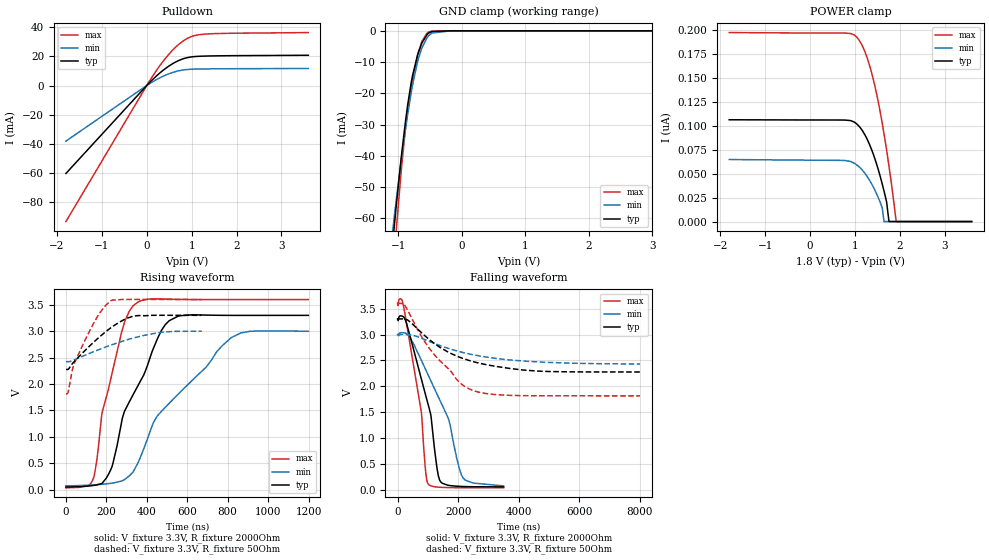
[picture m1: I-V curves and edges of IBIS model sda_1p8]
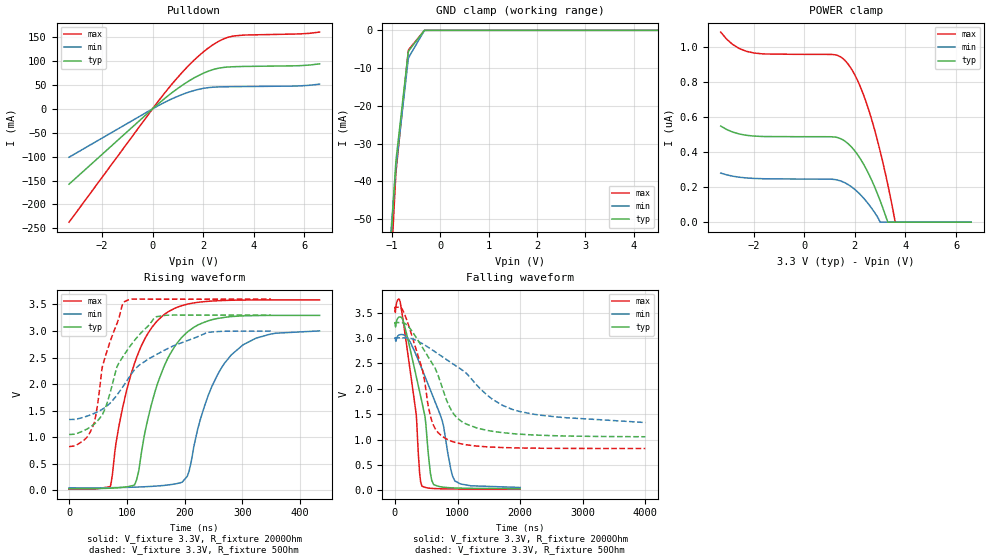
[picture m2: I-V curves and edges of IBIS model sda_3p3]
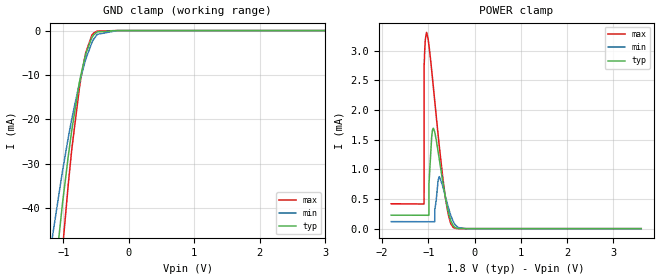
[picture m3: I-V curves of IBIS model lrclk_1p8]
|Texas Instruments Incorporated
| 2X50W/4Ohm PurePathTH Smart Amp
| Marketing part#   Voltage Range(Digital)   Package-type   #pins
| TAS5766MDCA   1.62V-3.6V   TSSOP   48
[IBIS Ver]   4.1
[File name]   tas5766m.ibs
[File Rev]   1.1
[Date]   01/23/2014
[Source]
| Texas Instruments Incorporated.
| Analog-eLab Design Center, HPA
| 12500 TI Blvd
| Dallas, TX -75243
[Notes]   Revision History:
| Rev 1.1: 01/23/2014
| - Updated ADR1 and ADR2 models
| Rev 1.0: 10/03/2013
| - Initial version of the model
| - Model generated from simulations in TISPICE
| - Model matched to SPICE simulation
| - Model names with a sda_1p8,lrclk_1p8,adr*_1p8 contain the models
|   for 1.8V (1.62V and 1.98V) operation.All other Model names with a trailing
|   _1p8 contains the model for 1.8V (1.65V and 1.95V) operation.
|   Model names with trailing _3p3contains the model for
|   3.3V (3.0V and 3.6V) operation.
| - Combined Pulldown/up non-monotonicity warnings for GPIO6_xxxx,
|   GPIO_xxxx. LRCK_xxxx reflect simulation results and can
|   safely ignored.
| - C_comp although listed in numerical order of value are
|   obtained from varying PVT conditions. For PVT conditions for
|   each specific value refer the buffer description under
|   respective [Model]. IBIS model user is responsible for using
|   appropriate C_comp to simulate for Signal Integrity.
|*EXCEPTION:   *
|* - For SDA and ADR2 models,There will be small leakage currents in   *
|* - POWER clamp IV-table because of the resistor (RES3T_NWELL) connected   *
|* - to the pad.   *
[Disclaimer]
| This model is designed as an aid for customers of Texas Instruments.
| TI and its licensors and suppliers make no warranties, either expressed
| or implied, with respect to this  model, including the warranties of
| merchantability or fitness for a particular purpose. The model is
| provided solely on an "as is" basis. The entire risk as to its quality
| and performance is with the customer.
[Copyright]
(C) Copyright 2014 Texas Instruments Incorporated.All rights reserved.
|   TAS5766MDCA
[Component]   TAS5766MDCA
[Manufacturer]   TI
[Package]   |48 TSSOP  -   package
|   typ   min   max
R_pkg   0.1   0.08   0.12
L_pkg   1.5nH   1.35nH   1.65nH
C_pkg   0.5pF   0.4pF   0.6pF
[Pin]  signal_name   model_name   R_pin   L_pin   C_pin
1   BSNR   NC   NA   NA   NA
2   OUTNR   NC   NA   NA   NA
3   GND   GND   NA   NA   NA
4   OUTPR   NC   NA   NA   NA
5   BSPR   NC   NA   NA   NA
6   PVCC   POWER   NA   NA   NA
7   PVCC   POWER   NA   NA   NA
8   GVDD   NC   NA   NA   NA
9   GAIN/FSW   NC   NA   NA   NA
10   GND   GND   NA   NA   NA
11   INNR   NC   NA   NA   NA
12   INPR   NC   NA   NA   NA
13   DACR   NC   NA   NA   NA
14   AVDD   POWER   NA   NA   NA
15   GND   GND   NA   NA   NA
16   SDA   SDA   NA   NA   NA
17   SCL   MC   NA   NA   NA
18   GPIO1   GPIO   NA   NA   NA
19   GPIO2   GPIO   NA   NA   NA
20   ADR2   ADR2   NA   NA   NA
21   GPIO3   GPIO6   NA   NA   NA
22   SCLK   SCK_IN   NA   NA   NA
23   BCLK   BCK_IN   NA   NA   NA
24   DIN   SCK_IN   NA   NA   NA
25   LRCLK   LRCLK   NA   NA   NA
26   ADR1   ADR1   NA   NA   NA
27   XSMT/UVP   DEMP_IN   NA   NA   NA
28   LDOO   NC   NA   NA   NA
29   GND   GND   NA   NA   NA
30   DVDD   POWER   NA   NA   NA
31   CPVDD   POWER   NA   NA   NA
32   CAPP   NC   NA   NA   NA
33   GND   GND   NA   NA   NA
34   CAPM   NC   NA   NA   NA
35   VNEG   NC   NA   NA   NA
36   DACL   NC   NA   NA   NA
37   INPL   NC   NA   NA   NA
38   INNL   NC   NA   NA   NA
39   GND   GND   NA   NA   NA
40   /FAULTZ   NC   NA   NA   NA
41   AVCC   POWER   NA   NA   NA
42   PVCC   POWER   NA   NA   NA
43   PVCC   POWER   NA   NA   NA
44   BSPL   NC   NA   NA   NA
45   OUTPL   NC   NA   NA   NA
46   GND   GND   NA   NA   NA
47   OUTNL   NC   NA   NA   NA
48   BSNL   NC   NA   NA   NA
|   Model Selectors
[Model Selector] SDA
sda_3p3   3.3V digital I/O_open_drain
sda_1p8   1.8V digital I/O_open_drain
[Model Selector] LRCLK
lrclk_3p3   3.3V digital input
lrclk_1p8   1.8V digital input
[Model Selector] ADR1
adr1_3p3   3.3V digital input
adr1_1p8   1.8V digital input
[Model Selector] ADR2
adr2_3p3   3.3V digital input
adr2_1p8   1.8V digital input
[Model Selector] MC
mc_3p3   3.3V digital input
mc_1p8   1.8V digital input
[Model Selector] GPIO
gpio_3p3   3.3V digital I/O
gpio_1p8   1.8V digital I/O
[Model Selector] GPIO6
gpio6_3p3   3.3V digital I/O
gpio6_1p8   1.8V digital I/O
[Model Selector] BCK_IN
bck_in_3p3   3.3V digital input
bck_in_1p8   1.8V digital input
[Model Selector] DEMP_IN
demp_in_3p3   3.3V digital input
demp_in_1p8   1.8V digital input
[Model Selector] FLT_IN
flt_in_3p3   3.3V digital input
flt_in_1p8   1.8V digital input
[Model Selector] SCK_IN
sck_in_3p3   3.3V digital input
sck_in_1p8   1.8V digital input
| Models and submodels in the file (22): sda_1p8 (I/O_open_drain), sda_3p3 (I/O_open_drain), lrclk_1p8 (Input), lrclk_3p3 (Input), adr1_1p8 (Input), adr1_3p3 (Input), adr2_1p8 (Input), adr2_3p3 (Input), mc_1p8 (Input), mc_3p3 (Input), gpio_1p8 (I/O), gpio_3p3 (I/O), gpio6_1p8 (I/O), gpio6_3p3 (I/O), bck_in_1p8 (Input), bck_in_3p3 (Input), demp_in_1p8 (Input), demp_in_3p3 (Input), flt_in_1p8 (Input), flt_in_3p3 (Input), sck_in_1p8 (Input), sck_in_3p3 (Input)
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|   sda_1p8 Model
[Model]   sda_1p8
Model_type   I/O_open_drain
Polarity   Non-Inverting
Vinl = 0.54
Vinh = 1.26
Vmeas = 0.9
Vref = 1.8
Cref = 400pF
Rref = 2000
|   typ   min   max
|   (nom PVT)   (fast PVT)   (slow PVT)
C_comp   1.016e-11   1.003e-11   1.042e-11
[Model spec]
|subparameter
Vinl   0.54   0.486   0.594
Vinh   1.26   1.134   1.386
| Where nom  PVT is Nominal Process, 1.8V, 27C
|   Fast PVT is Strong Process,  1.98V, -40C
|   Slow PVT is Weak Process,   1.62V, 125C
[Voltage Range]   1.8   1.62   1.98
|Junction Temperature
[Temperature Range]   27   125   -40
[Pullup Reference]   1.8   1.62   1.98
[Pulldown Reference]   0   0   0
[Power Clamp Reference]   1.8   1.62   1.98
[GND Clamp Reference]   0   0   0
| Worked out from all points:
|   slope of the pulldown table from 0 to 0.27 V, typ, clamps not added: 33.8 ohm
|   GND clamp passes 1 mA (typ) near -0.54 V on its own axis
|   falling waveform, V_fixture 3.3V, R_fixture 2000Ohm: 20-80 % time 682ns typ, 1.08us min, 481ns max; typ from 3.3 V to 0.054 V
|   rising waveform, V_fixture 3.3V, R_fixture 2000Ohm: 20-80 % time 185ns typ, 339ns min, 111ns max; typ from 0.051 V to 3.3 V
|   falling waveform, V_fixture 3.3V, R_fixture 50Ohm: 20-80 % time 1.78us typ, 2.22us min, 1.37us max; typ from 3.3 V to 2.28 V
|   rising waveform, V_fixture 3.3V, R_fixture 50Ohm: 20-80 % time 179ns typ, 257ns min, 124ns max; typ from 2.27 V to 3.3 V
[Pulldown]
|   Voltage   I(typ)   I(min)   I(max)
-1.8V     -60.2mA    -38.06mA   -93.14mA
113.4mV   3.549mA    2.205mA    5.58mA
290.9mV   8.545mA    5.245mA    13.57mA
466.2mV   12.73mA    7.698mA    20.46mA
597.4mV   15.29mA    9.13mA     24.88mA
790.2mV   18.06mA    10.53mA    30.04mA
1.022V    19.67mA    11.17mA    33.79mA
1.328V    20.17mA    11.36mA    35.25mA
3.6V      20.7mA     11.65mA    36.23mA
[GND Clamp]
|   Voltage   I(typ)   I(min)   I(max)
-1.8V     -334.9mA   -249.2mA   -436.8mA
-1.252V   -106.9mA   -94.42mA   -128.4mA
-1.061V   -62.46mA   -59.36mA   -71.93mA
-1.028V   -55.6mA    -53.82mA   -63.33mA
-943.2mV  -39.01mA   -40.16mA   -42.95mA
-880.3mV  -28.25mA   -30.88mA   -30.48mA
-795.8mV  -16.72mA   -19.9mA    -18.15mA
-696mV    -7.878mA   -9.987mA   -8.008mA
-627.4mV  -3.937mA   -5.498mA   -3.416mA
-518.4mV  -696.6uA   -1.541mA   -348.2uA
-180mV    -66.44nA   -964.8nA   -76.84nA
3.6V      0A         0A         0A
[POWER Clamp]
|   Voltage   I(typ)   I(min)   I(max)
-1.8V     106.1nA    64.68nA    197nA
732.5mV   105.9nA    63.75nA    196.5nA
1.004V    103.1nA    60.33nA    193.9nA
1.222V    90.44nA    50.33nA    177.2nA
1.328V    80.07nA    42.88nA    162.4nA
1.449V    64.89nA    32.34nA    140.4nA
1.607V    39.39nA    14.45nA    102.8nA
1.649V    31.66nA    0A         91.34nA
1.706V    20.31nA    0A         74.4nA
1.758V    0A         0A         57.99nA
1.919V    0A         0A         0A
3.6V      0A         0A         0A
[Ramp]
R_load = 2000
|   typ   min   max
dV/dt_r   1.94882/1.84537e-07   1.7551/3.39722e-07   2.13774/1.10149e-07
dV/dt_f   1.94589/6.79836e-07   1.72347/1.07088e-06   2.13801/4.80512e-07
[Falling Waveform]
V_fixture = 3.3V
V_fixture_min = 3V
V_fixture_max = 3.6V
R_fixture = 2000Ohm
|   Time   V(typ)   V(min)   V(max)
0s        3.3V       3V         3.6V
147.6ns   3.357V     3.036V     3.663V
300ns     3.202V     3.017V     3.201V
788.1ns   2.131V     2.498V     1.48V
908.8ns   1.865V     2.344V     456.9mV
996.5ns   1.673V     2.233V     121.6mV
1.419us   152.5mV    1.701V     45.98mV
1.684us   83.95mV    1.36V      40.46mV
2.172us   61.38mV    218.6mV    37.06mV
3.5us     54.21mV    73.33mV    35.56mV
[Rising Waveform]
V_fixture = 3.3V
V_fixture_min = 3V
V_fixture_max = 3.6V
R_fixture = 2000Ohm
|   Time   V(typ)   V(min)   V(max)
0s        50.87mV    74.1mV     35.46mV
135.6ns   80.3mV     91.04mV    212.9mV
178.9ns   122.3mV    103mV      1.462V
227.5ns   432.9mV    124mV      2.196V
279.8ns   1.365V     171.3mV    3.04V
335.8ns   1.824V     360.7mV    3.492V
472.6ns   3.016V     1.484V     3.609V
552.3ns   3.279V     1.796V     3.6V
864.3ns   3.298V     2.965V     3.597V
1.199us   3.299V     2.999V     3.598V
[Falling Waveform]
V_fixture = 3.3V
V_fixture_min = 3V
V_fixture_max = 3.6V
R_fixture = 50Ohm
|   Time   V(typ)   V(min)   V(max)
0s        3.3V       3V         3.6V
239.2ns   3.299V     3.001V     3.564V
801ns     3.029V     2.925V     2.951V
1.231us   2.82V      2.824V     2.597V
1.755us   2.636V     2.717V     2.29V
2.045us   2.562V     2.669V     2.074V
2.464us   2.48V      2.612V     1.923V
3.198us   2.388V     2.542V     1.84V
4.609us   2.294V     2.471V     1.816V
8us       2.276V     2.428V     1.814V
[Rising Waveform]
V_fixture = 3.3V
V_fixture_min = 3V
V_fixture_max = 3.6V
R_fixture = 50Ohm
|   Time   V(typ)   V(min)   V(max)
0s        2.275V     2.423V     1.814V
10.75ns   2.277V     2.423V     1.848V
31.25ns   2.383V     2.44V      2.259V
40.5ns    2.422V     2.455V     2.387V
87.75ns   2.609V     2.534V     2.776V
155.8ns   2.856V     2.64V      3.275V
219.5ns   3.057V     2.732V     3.571V
346.3ns   3.291V     2.883V     3.6V
480.5ns   3.3V       2.981V     3.6V
671.3ns   3.3V       3V         3.6V
|   sda_3p3 Model
[Model]   sda_3p3
Model_type   I/O_open_drain
Polarity   Non-Inverting
Vinl = 0.8
Vinh = 2
Vmeas = 1.65
Vref = 3.3
Cref = 400pF
Rref = 2000
|   typ   min   max
|   (nom PVT)   (fast PVT)   (slow PVT)
C_comp   9.904e-12   9.904e-12   1.003e-11
| Where nom  PVT is Nominal Process, 3.3V, 27C
|   Fast PVT is Strong Process,  3.6V, -40C
|   Slow PVT is Weak Process,   3V, 125C
[Voltage Range]   3.3   3   3.6
|Junction Temperature
[Temperature Range]   27   125   -40
[Pullup Reference]   3.3   3   3.6
[Pulldown Reference]   0   0   0
[Power Clamp Reference]   3.3   3   3.6
[GND Clamp Reference]   0   0   0
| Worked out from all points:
|   slope of the pulldown table from 0 to 0.495 V, typ, clamps not added: 22.1 ohm
|   falling waveform, V_fixture 3.3V, R_fixture 2000Ohm: 20-80 % time 268ns typ, 434ns min, 189ns max; typ from 3.3 V to 0.036 V
|   rising waveform, V_fixture 3.3V, R_fixture 2000Ohm: 20-80 % time 54.2ns typ, 57.3ns min, 52.8ns max; typ from 0.035 V to 3.29 V
|   falling waveform, V_fixture 3.3V, R_fixture 50Ohm: 20-80 % time 518ns typ, 1.02us min, 316ns max; typ from 3.3 V to 1.06 V
|   rising waveform, V_fixture 3.3V, R_fixture 50Ohm: 20-80 % time 54.4ns typ, 96.8ns min, 33.8ns max; typ from 1.05 V to 3.3 V
[Pulldown]
|   Voltage   I(typ)   I(min)   I(max)
-3.3V     -157.6mA   -101.2mA   -237.1mA
459mV     20.85mA    13.12mA    31.8mA
897mV     38.95mA    24.09mA    59.96mA
1.434V    58.29mA    35.03mA    91.05mA
2.172V    78.17mA    44.18mA    126mA
2.442V    82.93mA    45.46mA    136mA
2.806V    86.68mA    46.14mA    146.3mA
3.231V    88.2mA     46.48mA    152.6mA
5.625V    90.03mA    47.68mA    156.5mA
6.6V      94.16mA    51.61mA    160.6mA
[GND Clamp]
|   Voltage   I(typ)   I(min)   I(max)
-3.3V     -1.594A    -1.313A    -1.903A
-1.104V   -71.9mA    -66.9mA    -83.83mA
-927mV    -36.1mA    -37.7mA    -39.48mA
-916.8mV  -34.31mA   -36.17mA   -37.38mA
-666.6mV  -6.007mA   -7.839mA   -5.788mA
-657.6mV  -5.489mA   -7.251mA   -5.183mA
-330mV    -4.474uA   -40.92uA   -707.9nA
6.6V      0A         0A         0A
[POWER Clamp]
|   Voltage   I(typ)   I(min)   I(max)
-3.3V     548.4nA    280.3nA    1.085uA
-2.828V   514.4nA    262.6nA    1.014uA
-1.986V   491.3nA    249.7nA    965.5nA
1.096V    487.3nA    245.1nA    957nA
1.53V     469.6nA    230.1nA    933.6nA
2.046V    397.8nA    181.1nA    827.2nA
2.303V    341.4nA    144.3nA    741.6nA
2.571V    268.7nA    97.75nA    630.3nA
3.003V    121.8nA    0A         404.4nA
3.303V    0A         0A         214.2nA
3.598V    0A         0A         0A
6.6V      0A         0A         0A
[Ramp]
R_load = 2000
|   typ   min   max
dV/dt_r   1.95666/5.39715e-08   1.76885/5.68771e-08   2.14112/5.31045e-08
dV/dt_f   1.9577/2.68023e-07   1.7646/4.3247e-07   2.14366/1.89177e-07
[Falling Waveform]
V_fixture = 3.3V
V_fixture_min = 3V
V_fixture_max = 3.6V
R_fixture = 2000Ohm
|   Time   V(typ)   V(min)   V(max)
0s        3.299V     3V         3.598V
68.6ns    3.411V     3.06V      3.763V
113ns     3.393V     3.067V     3.495V
340.9ns   2.244V     2.66V      1.492V
394.8ns   1.944V     2.501V     344.9mV
430.8ns   1.744V     2.393V     85.5mV
566.9ns   341mV      1.975V     42.72mV
619.3ns   114.8mV    1.813V     37.98mV
958.5ns   48.99mV    186.8mV    28.49mV
2us       36.19mV    58.51mV    25.32mV
[Rising Waveform]
V_fixture = 3.3V
V_fixture_min = 3V
V_fixture_max = 3.6V
R_fixture = 2000Ohm
|   Time   V(typ)   V(min)   V(max)
0s        34.62mV    49.13mV    25.01mV
71.2ns    43.01mV    52.36mV    71.31mV
86.2ns    53.37mV    55.49mV    1.207V
113.4ns   103.5mV    63.17mV    2.394V
142.3ns   1.606V     77.4mV     3.051V
164.5ns   2.336V     95.49mV    3.309V
204.5ns   2.979V     265.2mV    3.506V
241ns     3.193V     1.792V     3.56V
280.7ns   3.273V     2.551V     3.58V
433.6ns   3.295V     3.003V     3.586V
[Falling Waveform]
V_fixture = 3.3V
V_fixture_min = 3V
V_fixture_max = 3.6V
R_fixture = 50Ohm
|   Time   V(typ)   V(min)   V(max)
0s        3.3V       3V         3.6V
111.2ns   3.303V     3.002V     3.581V
221.2ns   3.218V     2.997V     3.239V
442.8ns   2.808V     2.885V     2.361V
532.8ns   2.626V     2.816V     1.664V
603ns     2.485V     2.76V      1.317V
817ns     1.801V     2.581V     1.017V
1.094us   1.335V     2.352V     908mV
1.875us   1.118V     1.594V     838.7mV
4us       1.056V     1.336V     825.3mV
[Rising Waveform]
V_fixture = 3.3V
V_fixture_min = 3V
V_fixture_max = 3.6V
R_fixture = 50Ohm
|   Time   V(typ)   V(min)   V(max)
0s        1.053V     1.336V     825.1mV
28.8ns    1.144V     1.391V     978.1mV
43.8ns    1.25V      1.451V     1.282V
58ns      1.432V     1.531V     2.343V
83ns      2.328V     1.797V     3.142V
96ns      2.565V     1.997V     3.554V
114.8ns   2.845V     2.293V     3.602V
151ns     3.27V      2.557V     3.6V
239.8ns   3.3V       2.976V     3.6V
349.6ns   3.3V       3V         3.6V
|   lrclk_1p8 Model
[Model]   lrclk_1p8
Model_type   Input
Vinl = 0.54
Vinh = 1.26
|   typ   min   max
|   (nom PVT)   (fast PVT)   (slow PVT)
C_comp   6.878e-12   6.276e-12   7.174e-12
[Model spec]
|subparameter
Vinl   0.54   0.486   0.594
Vinh   1.26   1.134   1.386
| Where nom  PVT is Nominal Process, 1.8V, 27C
|   Fast PVT is Strong Process,  1.98V, -40C
|   Slow PVT is Weak Process,   1.62V, 125C
[Voltage Range]   1.8   1.62   1.98
|Junction Temperature
[Temperature Range]   27   125   -40
[Power Clamp Reference]   1.8   1.62   1.98
[GND Clamp Reference]   0   0   0
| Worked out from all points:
|   GND clamp passes 1 mA (typ) near -0.54 V on its own axis
|   POWER clamp passes 1 mA (typ) near -0.73 V on its own axis
[GND Clamp]
|   Voltage   I(typ)   I(min)   I(max)
-1.8V     -274mA     -172mA     -383.3mA
-1.162V   -59.61mA   -45.98mA   -78.12mA
-1.013V   -38.93mA   -31.66mA   -49.29mA
-925.2mV  -28.28mA   -24.11mA   -34.63mA
-869.4mV  -22.23mA   -19.73mA   -26.46mA
-736.2mV  -10.28mA   -10.66mA   -11.09mA
-657.5mV  -5.238mA   -6.396mA   -4.955mA
-564.5mV  -1.563mA   -2.689mA   -1.03mA
-538.2mV  -983.7uA   -1.952mA   -555.3uA
-481.3mV  -292.5uA   -842.1uA   -114uA
-180mV    -19.95nA   -834.7nA   0A
3.6V      0A         0A         0A
[POWER Clamp]
|   Voltage   I(typ)   I(min)   I(max)
-1.8V     227.8uA    118.2uA    419.5uA
-1.091V   226uA      117.3uA    415.4uA
-1.089V   226uA      117.3uA    2.738mA
-1.038V   225.9uA    117.3uA    3.308mA
-986.4mV  225.4uA    117.2uA    3.099mA
-984.6mV  748.8uA    117.2uA    3.088mA
-927mV    1.535mA    117.1uA    2.677mA
-891mV    1.692mA    117uA      2.396mA
-761.6mV  1.17mA     876.6uA    1.388mA
-617.4mV  473.3uA    505uA      458.3uA
-461.5mV  50.53uA    122.7uA    23.06uA
3.6V      0A         0A         0A
